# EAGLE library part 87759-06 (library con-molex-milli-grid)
HEADER
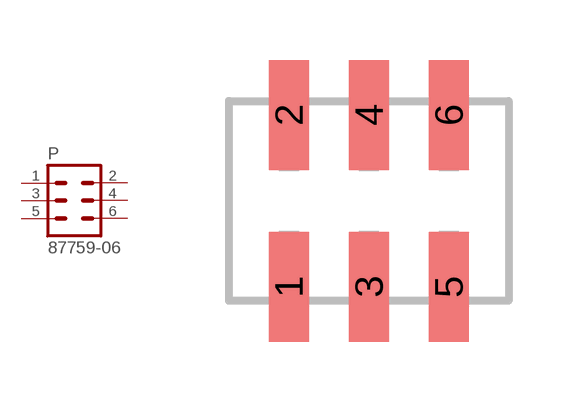
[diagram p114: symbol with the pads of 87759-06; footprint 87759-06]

Designator prefix P

## 87759-06  [87759-06]
1  1  pas
2  2  pas
3  3  pas
4  4  pas
5  5  pas
6  6  pas

## Footprint 87759-06 (pad centres in mm)
HEADER SMD Dual Row, Vertical
smd 1 x 2.75: 1 -2,-2.15; 2 -2,2.15; 3 0,-2.15; 4 0,2.15; 5 2,-2.15; 6 2,2.15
